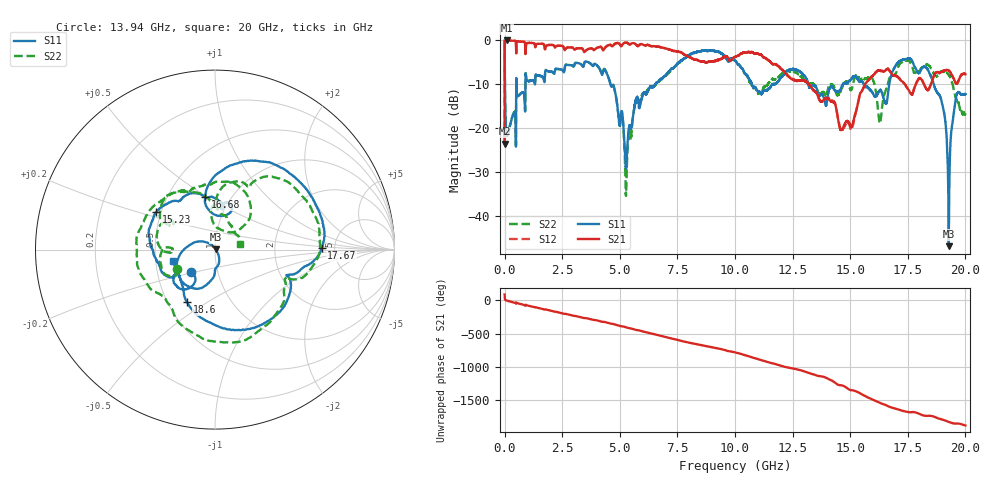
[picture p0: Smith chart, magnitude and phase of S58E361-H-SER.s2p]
!{S58E361}
!Johanson Technology Inc.
!www.johansontechnology.com
!Test Board Conditions:
!Substrate Type  RO4350B
!Substrate Thickness  60 mil
!Substrate Dk  3.66
!TL Type: GCPW
!TL Trace Width  115 mil
!TL Gap  52 mil
!Electrode orientation  Horizontal
!DUT TOPOLOGY	SERIES
!Mounting Pad LxW  55x428 mil
! Created Wed Apr 14 11:45:08 2021
# mhz S ma R 50
! 2 Port Network Data from SP1.SP block
! freq  magS11  angS11  magS21  angS21  magS12  angS12  magS22  angS22
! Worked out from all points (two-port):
!   20001 points, 300 kHz to 20 GHz, reference 50 ohm
!   highest |S21| = -0.03 dB at 100.3 MHz (marker M1); lowest = -23.6 dB at 300 kHz (marker M2)
!   |S21| within 3 dB of the highest: 4.492 MHz to 901.9 MHz (897.4 MHz wide, 198 % of centre); 905.8 MHz to 7.737 GHz (6.831 GHz wide, 158 % of centre)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
!   lowest |S11| = -47.0 dB at 19.28 GHz (marker M3), VSWR 1.01, Z = 50.4 + j0.161 ohm
!   |S11| at or under -10 dB: 4.594 GHz to 6.548 GHz (1.953 GHz wide, 35.1 % of centre); 13.18 GHz to 14.69 GHz (1.506 GHz wide, 10.8 % of centre); 18.63 GHz to end of sweep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
!   |S22| runs from -35.5 to -0.1 dB; largest |S21 - S12| = 0.012
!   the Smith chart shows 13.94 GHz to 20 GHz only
!   S11 on the Smith chart (normalised r, x): 13.94 GHz: 0.75, -0.19; 15.23 GHz: 0.47, +0.23; 16.68 GHz: 0.76, +0.49; 17.67 GHz: 3.92, +0.08; 18.6 GHz: 0.63, -0.41; 20 GHz: 0.62, -0.08
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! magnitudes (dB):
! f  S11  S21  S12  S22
! 300 kHz  -0.1  -23.6  -23.5  -0.1
! 100.3 MHz  -21.8  0.0  0.0  -21.7
! 1.001 GHz  -9.3  -0.6  -0.6  -9.2
! 3.334 GHz  -5.5  -1.8  -1.8  -5.5
! 4.726 GHz  -10.3  -1.1  -1.1  -10.3
! 5.276 GHz  -29.0  -0.5  -0.5  -34.5
! 5.683 GHz  -13.9  -0.9  -0.9  -14.1
! 6.667 GHz  -9.5  -1.4  -1.5  -9.6
! 10 GHz  -4.6  -3.8  -3.8  -4.7
! 13.33 GHz  -10.5  -10.9  -10.8  -9.7
! 13.94 GHz  -14.9  -13.3  -13.1  -12.5
! 15.23 GHz  -8.2  -16.6  -16.8  -8.1
! 15.95 GHz  -11.8  -8.2  -8.2  -8.7
! 16.29 GHz  -11.4  -6.9  -6.9  -18.8
! 16.67 GHz  -11.0  -6.6  -6.7  -9.3
! 16.68 GHz  -10.5  -6.7  -6.8  -9.0
! 17.67 GHz  -4.5  -12.4  -12.2  -5.6
! 18.6 GHz  -9.6  -8.5  -8.5  -7.2
! 19.05 GHz  -15.8  -7.0  -7.0  -7.2
! 19.28 GHz  -47.0  -6.9  -6.8  -7.9
! 19.6 GHz  -12.9  -9.9  -9.8  -13.4
! 20 GHz  -12.3  -7.7  -7.7  -17.0
